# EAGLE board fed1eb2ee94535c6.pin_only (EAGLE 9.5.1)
REV: B

Size 50.8 x 22.86 mm. Coordinates in mm from the lower left corner, seen from the top.
Outline: 2.54,22.86 48.26,22.86 arc-90 50.8,20.32 50.8,2.54 arc-90 48.26,0 2.54,0 arc-90 0,2.54 0,9.14 0.51,9.65 0.51,13.21 0,13.72 0,20.32 arc-90 2.54,22.86
Copper layers (1+2*15+16): Top 0.035mm / dielectric 0.2mm / Route2 0.035mm / dielectric 1.45mm / Route15 0.035mm / dielectric 0.2mm / Bottom 0.035mm
Design rules "adafruit_4layer *": minimum track width 7mil, minimum drill 15.5mil, track to track 8mil, track to pad 8mil, pad to pad 8mil, via to via 8mil, smd to smd 8mil, copper to edge 10mil, drill to drill 8mil, minimum pad ring 10mil, minimum via ring 8mil, stop-mask expansion 2mil, vias tented up to drill 20mil, thermal gap 10mil
Net classes: 1 power: width 0.254 mm

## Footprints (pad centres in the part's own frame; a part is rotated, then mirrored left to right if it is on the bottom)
0603-NO = smd 1.075 x 1: 1 -0.85,0; 2 0.85,0
0805-NO = smd 1.24 x 1.5: 1 -0.95,0; 2 0.95,0
SOD-123 = smd 1.4 x 1.4: A 1.85,0; C -1.85,0
CHIPLED_0805_NOOUTLINE = smd 1.2 x 1.2: A 0,-1.05; C 0,1.05
CHIPLED_0603_NOOUTLINE = smd 0.8 x 0.8: A 0,-0.75; C 0,0.75
TP10R = smd 1 x 1: TP 0,0
FIDUCIAL_1MM = smd 1 x 1: 1 0,0
LGA16_3X3MM = smd 0.5 x 0.25: 1 -1.35,1; 2 -1.35,0.5; 3 -1.35,0; 4 -1.35,-0.5; 5 -1.35,-1; 9 1.35,-1; 10 1.35,-0.5; 11 1.35,0; 12 1.35,0.5; 13 1.35,1 | smd 0.25 x 0.5: 6 -0.5,-1.35; 7 0,-1.35; 8 0.5,-1.35; 14 0.5,1.35; 15 0,1.35; 16 -0.5,1.35
USON8 = smd 0.5 x 0.275: 1 -1.2,0.75; 2 -1.2,0.25; 3 -1.2,-0.25; 4 -1.2,-0.75; 5 1.2,-0.75; 6 1.2,-0.25; 7 1.2,0.25; 8 1.2,0.75
LGA12_2X2MM = smd 0.275 x 0.25: 1 -0.75,0.75; 2 -0.75,0.25; 3 -0.75,-0.25; 4 -0.75,-0.75; 7 0.75,-0.75; 8 0.75,-0.25; 9 0.75,0.25; 10 0.75,0.75 | smd 0.25 x 0.275: 5 -0.25,-0.75; 6 0.25,-0.75; 11 0.25,0.75; 12 -0.25,0.75
SPK0415HM4H = smd 0.45 x 0.95: 1 0.425,-0.625; 2 0.425,0.625; 3 -0.425,0.625; 4 -0.425,-0.625 | smd 1.2 x 0.45: 5 0,-1.75; 7 0,1.75 | smd 0.45 x 2.2: 6 1.25,0; 8 -1.25,0
_0805MP = smd 1.2 x 1.3: 1 -1.016,0; 2 1.016,0
LED3535 = smd 1 x 0.85: 1 -1.75,0.875; 2 -1.75,-0.875; 3 1.75,-0.875; 4 1.75,0.875
MDBT50 = smd 0.6 x 0.4: 1 -4.65,3.75; 2 -4.65,2.65; 3 -4.65,1.85; 4 -4.65,0.25; 5 -3.75,-0.15; 6 -4.65,-0.55; 7 -3.75,-0.95; 8 -4.65,-1.35; 9 -3.75,-1.75; 10 -4.65,-2.15; 11 -3.75,-2.55; 12 -4.65,-2.95; 13 -3.75,-3.35; 14 -4.65,-3.75; 34 4.65,-6.15; 35 4.65,-5.35; 36 3.75,-4.95; 37 4.65,-4.55; 38 3.75,-4.15; 39 4.65,-3.75; 40 3.75,-3.35; 41 4.65,-2.95; 42 3.75,-2.55; 43 3.75,-1.75; 44 4.65,-1.35; 45 3.75,-0.95; 46 4.65,-0.55; 47 3.75,-0.15; 48 4.65,0.25; 49 3.75,0.65; 50 3.75,1.45; 51 4.65,1.85; 52 3.75,2.25; 53 4.65,2.65; 54 3.75,3.05; 55 4.65,3.75 | smd 0.4 x 0.6: 15 -4.8,-7.15; 16 -4,-7.15; 17 -3.2,-7.15; 18 -2.4,-7.15; 19 -2,-6.25; 20 -1.6,-7.15; 21 -1.2,-6.25; 22 -0.8,-7.15; 23 -0.4,-6.25; 24 0,-7.15; 25 0.4,-6.25; 26 0.8,-7.15; 27 1.2,-6.25; 28 1.6,-7.15; 29 2,-6.25; 30 2.4,-7.15; 31 3.2,-7.15; 32 4,-7.15; 33 4.8,-7.15; 56 -2,-0.55; 57 -1.2,-0.55; 58 -0.4,-0.55; 59 0.4,-0.55; 60 1.2,-0.55; 61 2,-0.55
FEATHERWING_NODIM = drill 1 pad 1.778: 1 6.35,1.27; 2 8.89,1.27; 3 11.43,1.27; 4 13.97,1.27; 5 16.51,1.27; 6 19.05,1.27; 7 21.59,1.27; 8 24.13,1.27; 9 26.67,1.27; 10 29.21,1.27; 11 31.75,1.27; 12 34.29,1.27; 13 36.83,1.27; 14 39.37,1.27; 15 41.91,1.27; 16 44.45,1.27; 17 44.45,21.59; 18 41.91,21.59; 19 39.37,21.59; 20 36.83,21.59; 21 34.29,21.59; 22 31.75,21.59; 23 29.21,21.59; 24 26.67,21.59; 25 24.13,21.59; 26 21.59,21.59; 27 19.05,21.59; 28 16.51,21.59 | drill 2.5 pad 3.81: P$1 2.54,20.32; P$2 2.54,2.54 | hole 2.54: 48.26,20.32; 48.26,2.54
SOT23-R = smd 0.635 x 1.016: 1 -0.95,-1; 2 0.95,-1; 3 0,1
RESPACK_4X0603 = smd 0.45 x 0.9: 1 -1.3,-0.85; 2 -0.4,-0.85; 3 0.4,-0.85; 4 1.3,-0.85; 5 1.3,0.85; 6 0.4,0.85; 7 -0.4,0.85; 8 -1.3,0.85
BTN_KMR2_4.6X2.8 = smd 0.9 x 0.9: A 2.05,0.8; A' -2.05,0.8; B 2.05,-0.8; B' -2.05,-0.8
TP12R = smd 1.2 x 1.2: TP 0,0
APDS-9960 = smd 0.6 x 0.72: 1 0.7,1.505; 2 0.7,0.505; 3 0.7,-0.495; 4 0.7,-1.495; 5 -0.7,-1.495; 6 -0.7,-0.495; 7 -0.7,0.505; 8 -0.7,1.505
SOT23-5 = smd 0.55 x 1.2: 1 -0.95,-1.3; 2 0,-1.3; 3 0.95,-1.3; 4 0.95,1.3; 5 -0.95,1.3
SHT3X = smd 0.6 x 0.25: 1 -1.15,0.75; 2 -1.15,0.25; 3 -1.15,-0.25; 4 -1.15,-0.75; 5 1.15,-0.75; 6 1.15,-0.25; 7 1.15,0.25; 8 1.15,0.75 | smd 1 x 1.7: THERMAL 0,0
BMP280 = smd 0.5 x 0.35: 1 0.8,0.975; 2 0.8,0.325; 3 0.8,-0.325; 4 0.8,-0.975; 5 -0.8,-0.975; 6 -0.8,-0.325; 7 -0.8,0.325; 8 -0.8,0.975
4UCONN_20329_V2 = smd 1 x 2: BASE@1 -0.75,-2; BASE@2 0.75,-2 | smd 0.4 x 1.35: D+ 0,0.775; D- -0.65,0.775; GND 1.3,0.775; ID 0.65,0.775; VBUS -1.3,0.775 | drill 0.8 pad 1.143 offset: SPRT@1 -3.3,0.9; SPRT@2 3.3,0.9 | drill 0.9 pad 2.413 square: SPRT@3 -3.6,-1.9; SPRT@4 3.6,-1.9 | hole 0.7: -1.95,0; 1.95,0
JSTPH2 = smd 1 x 4.6: 1 -1,-3.7; 2 1,-3.7 | smd 1.6 x 3.4: NC1 -3.4,1.5; NC2 3.4,1.5

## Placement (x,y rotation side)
C1  0.1uF  [0603-NO]  24.83,17.21 270 top
C3  0.1uF  [0603-NO]  19.08,8.79 0 top
C4  1uF  [0603-NO]  31.31,10.2 0 top
C5  10uF  [0805-NO]  18.8,10.38 0 top
C6  10uF  [0805-NO]  21.08,17.91 180 top
C7  10uF  [0805-NO]  12.29,9.86 90 top
C8  10uF  [0805-NO]  31.31,8.71 0 top
C9  10uF  [0805-NO]  15.32,12.26 180 top
C10  0.1uF  [0603-NO]  33.27,16.64 90 top
C12  0.1uF  [0603-NO]  26.16,17.21 270 top
C13  0.1uF  [0603-NO]  31.31,11.49 0 top
D1  MBR054  [SOD-123]  10.26,12.4 180 top
D2  RED  [CHIPLED_0805_NOOUTLINE]  2.22,17.27 90 top
D3  ORANGE  [CHIPLED_0805_NOOUTLINE]  2.08,5.64 270 top
D4  BLUE  [CHIPLED_0603_NOOUTLINE]  45.34,18.03 180 top
D+  TPTP10R  [TP10R]  5.46,10.79 0 bottom
D-  TPTP10R  [TP10R]  5.46,12 0 bottom
FID1  FIDUCIAL_1MM  [FIDUCIAL_1MM]  10.67,21.84 0 top
FID2  FIDUCIAL_1MM  [FIDUCIAL_1MM]  49.78,4.51 0 top
IC1  LSM6DS33  [LGA16_3X3MM]  22.42,14.54 90 top
IC2  GD25Q16  [USON8]  40.77,4.95 180 top
IC3  LIS3MDL  [LGA12_2X2MM]  25.84,13.4 180 top
IC4  MIC_PDM  [SPK0415HM4H]  30.54,17.27 90 top
L1  DNP  [_0805MP]  33.82,9.37 270 top
LED1  WS2812B3535  [LED3535]  19.39,6.15 180 top
MDBT1  MDBT50  [MDBT50]  42.55,11.43 270 top
MS1  FEATHERWING_NODIM  [FEATHERWING_NODIM]  0,0 0 top
Q3  DMG2305  [SOT23-R]  9.82,9.55 0 top
R1  2.2K  [0603-NO]  5.71,19.68 270 top
R3  1K  [0603-NO]  6.76,7.38 90 top
R4  4.7K  [0603-NO]  15.32,5.31 0 top
R7  4.7K  [RESPACK_4X0603]  42.61,18.22 180 top
R10  22  [0603-NO]  35.88,5.4 0 top
R11  22  [0603-NO]  36.83,4.13 0 top
R12  100K  [RESPACK_4X0603]  17.37,17.5 180 top
SW1  KMR2  [BTN_KMR2_4.6X2.8]  11.1,6.22 0 top
SW2  KMR2  [BTN_KMR2_4.6X2.8]  29.93,5.85 0 top
SWC  TPTP12R  [TP12R]  40.2,9.78 0 bottom
SWD  TPTP12R  [TP12R]  41.81,8.71 0 bottom
TP1  TPTP10R  [TP10R]  44.01,10.03 0 bottom
U1  APDS-9960  [APDS-9960]  26.35,10.22 90 top
U2  AP2112(3.3V)  [SOT23-5]  18.78,13.39 180 top
U3  MCP73831T-2ACI/OT  [SOT23-5]  15.14,9.14 180 top
U4  SHT30  [SHT3X]  22.48,10.67 0 top
U5  BMP280  [BMP280]  23.24,6.99 180 top
U$10  [PCBFEAT-REV-056]  44.43,5.64 0 bottom
U$14  [FEATHERSENSE_TOP]  0,0 0 top
U$75  [FEATHERSENSE_BOT]  50.8,0 0 bottom
X1  4u20329  [4UCONN_20329_V2]  4.45,11.43 270 top
X2  CON_JST_PH_2PIN_MTPH2  [JSTPH2]  10.79,19.3 0 top

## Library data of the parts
C1 C3-C10 C12 C13 D1-D4 IC2 IC4 L1 LED1 MDBT1 MS1 Q3 R1 R3 R4 R7 R10-R12 SW1 SW2 U2-U4 U$10 X1 X2 = microbuilder
D+ D- SWC SWD TP1 = testpad
FID1 FID2 = microbuilder; BOM: EXCLUDE
IC1 IC3 U1 U5 = adafruit_sensor
U$14 U$75 = feather_silks

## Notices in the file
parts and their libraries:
microbuilder: This work is placed in the public domain, and may be freely used for commercial and non-commercial work with the following conditions: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
